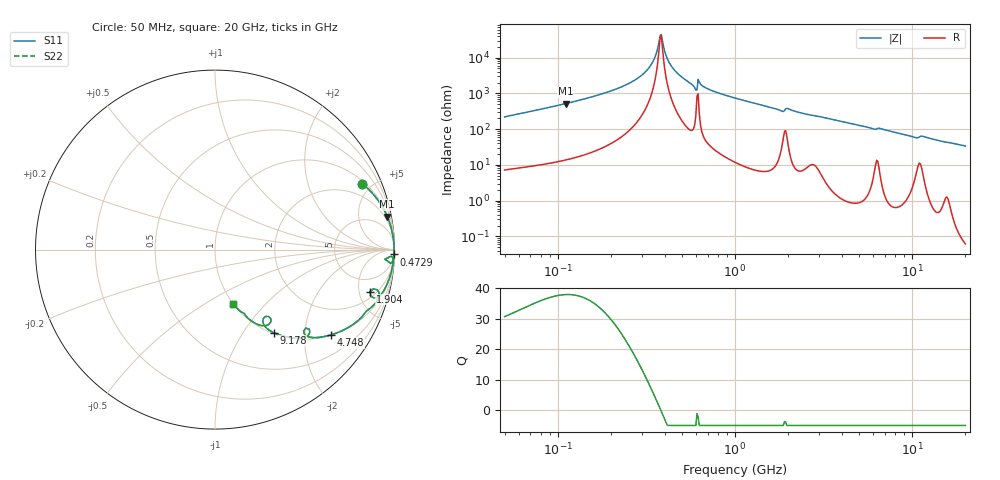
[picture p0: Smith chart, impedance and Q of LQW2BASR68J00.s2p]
!Murata Part Number: LQW2BASR68J00
!These Parameters are Measured in Series Mode Connection
!  o--[Z]--o
!Port1  Port2
!  o-------o
!Freq. Start=50[MHz] Stop=20[GHz], 401[Steps]
# Hz S RI R 50
!Freq.(Hz) S11(Real) S11(Imag) S21(Real) S21(Imag) S12(Real) S12(Imag) S22(Real) S22(Imag)
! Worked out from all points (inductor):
!   401 points, 50 MHz to 20 GHz, reference 50 ohm
!   read as one part in series: L = 685 nH near 51.52 MHz
!   highest Q = 37.9 at 110.6 MHz (marker M1), where L = 745 nH
!   self-resonance near 377.7 MHz
!   S11 on the Smith chart (normalised r, x): 50 MHz: 1.14, +4.40; 472.9 MHz: 7, -73; 1.904 GHz: 2.72, -6.37; 4.748 GHz: 1.02, -2.72; 9.178 GHz: 1.02, -1.38; 20 GHz: 1.00, -0.67
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5e7  0.8211 0.3673  0.1789 -0.3673  0.1789 -0.3673  0.8211 0.3673
1.105969e8  0.9595 0.1844  0.0405 -0.1844  0.0405 -0.1844  0.9595 0.1844
1.364002e8  0.9744 0.1449  0.0256 -0.1449  0.0256 -0.1449  0.9744 0.1449
2.170075e8  0.992 0.0722  0.00796 -0.0722  0.00796 -0.0722  0.992 0.0722
2.884513e8  0.9965 0.0346  0.00353 -0.0346  0.00353 -0.0346  0.9965 0.0346
3.401177e8  0.9976 0.0141  0.00239 -0.0141  0.00239 -0.0141  0.9976 0.0141
3.557498e8  0.9978 0.00853  0.00224 -0.00853  0.00224 -0.00853  0.9978 0.00853
3.721004e8  0.9978 0.00299  0.00215 -0.00299  0.00215 -0.00299  0.9978 0.00299
3.777159e8  0.9979 0.00114  0.00214 -0.00114  0.00214 -0.00114  0.9979 0.00114
3.892024e8  0.9979 -0.00256  0.00213 0.00256  0.00213 0.00256  0.9979 -0.00256
4.194704e8  0.9978 -0.0119  0.00224 0.0119  0.00224 0.0119  0.9978 -0.0119
4.728708e8  0.9972 -0.0272  0.00283 0.0272  0.00283 0.0272  0.9972 -0.0272
5.919973e8  0.9892 -0.0674  0.0108 0.0674  0.0108 0.0674  0.9892 -0.0674
6.380365e8  0.9931 -0.054  0.00694 0.054  0.00694 0.054  0.9931 -0.054
7.192613e8  0.9917 -0.0781  0.0083 0.0781  0.0083 0.0781  0.9917 -0.0781
1e9  0.98 -0.1321  0.02 0.1321  0.02 0.1321  0.98 -0.1321
1.904239e9  0.8633 -0.2341  0.1367 0.2341  0.1367 0.2341  0.8633 -0.2341
2.728004e9  0.8451 -0.3414  0.1549 0.3414  0.1549 0.3414  0.8451 -0.3414
4.748272e9  0.6483 -0.4744  0.3517 0.4744  0.3517 0.4744  0.6483 -0.4744
7.442007e9  0.4397 -0.492  0.5603 0.492  0.5603 0.492  0.4397 -0.492
9.178299e9  0.3262 -0.462  0.6738 0.462  0.6738 0.462  0.3262 -0.462
2e10  0.1017 -0.3014  0.8983 0.3014  0.8983 0.3014  0.1017 -0.3014
